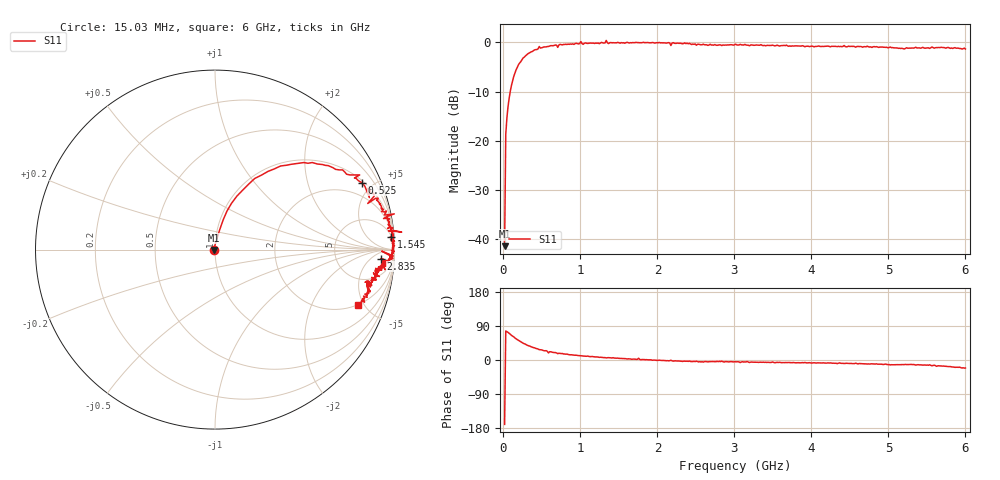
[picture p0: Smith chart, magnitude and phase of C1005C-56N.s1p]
!	Network	Analyzer	HP8753E.07.74:	Oct	30	2002	Serial	No.	JP38451487
!	Hewlett-Packard
!	7	Sep	2009	9:12:18
!	Frequency	S11
#	HZ	S	RI	R	50
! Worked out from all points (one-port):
!   400 points, 15.03 MHz to 6 GHz, reference 50 ohm
!   lowest |S11| = -41.4 dB at 15.03 MHz (marker M1), VSWR 1.02, Z = 49.2 - j0.147 ohm
!   |S11| at or under -10 dB: start of sweep to 88.39 MHz
!   S11 on the Smith chart (normalised r, x): 15.03 MHz: 0.98, -0.00; 525 MHz: 1.12, +4.32; 1.545 GHz: 5, +27; 2.835 GHz: 18, -12; 6 GHz: 1.97, -4.52
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1.502992e7  -0.00835 -0.00149
3.002985e7  0.027 0.113
6.00297e7  0.0664 0.214
9.002955e7  0.122 0.298
1.650292e8  0.296 0.436
2.550287e8  0.495 0.485
4.650277e8  0.806 0.416
5.250274e8  0.817 0.373
5.850271e8  0.86 0.29
6.150269e8  0.86 0.342
7.650262e8  0.9 0.277
1.005025e9  0.999 0.199
1.035025e9  0.939 0.173
1.245024e9  0.962 0.117
1.335023e9  1.04 0.0975
1.365023e9  0.966 0.105
1.515022e9  0.977 0.0717
1.545022e9  0.983 0.0706
1.755021e9  0.99 0.0818
2.145019e9  0.992 -0.0367
2.175019e9  0.929 -0.00864
2.265019e9  0.982 -0.0444
2.835016e9  0.925 -0.0497
3.015015e9  0.954 -0.0811
3.765011e9  0.91 -0.106
4.515007e9  0.9 -0.142
5.265004e9  0.853 -0.181
6e9  0.797 -0.309
